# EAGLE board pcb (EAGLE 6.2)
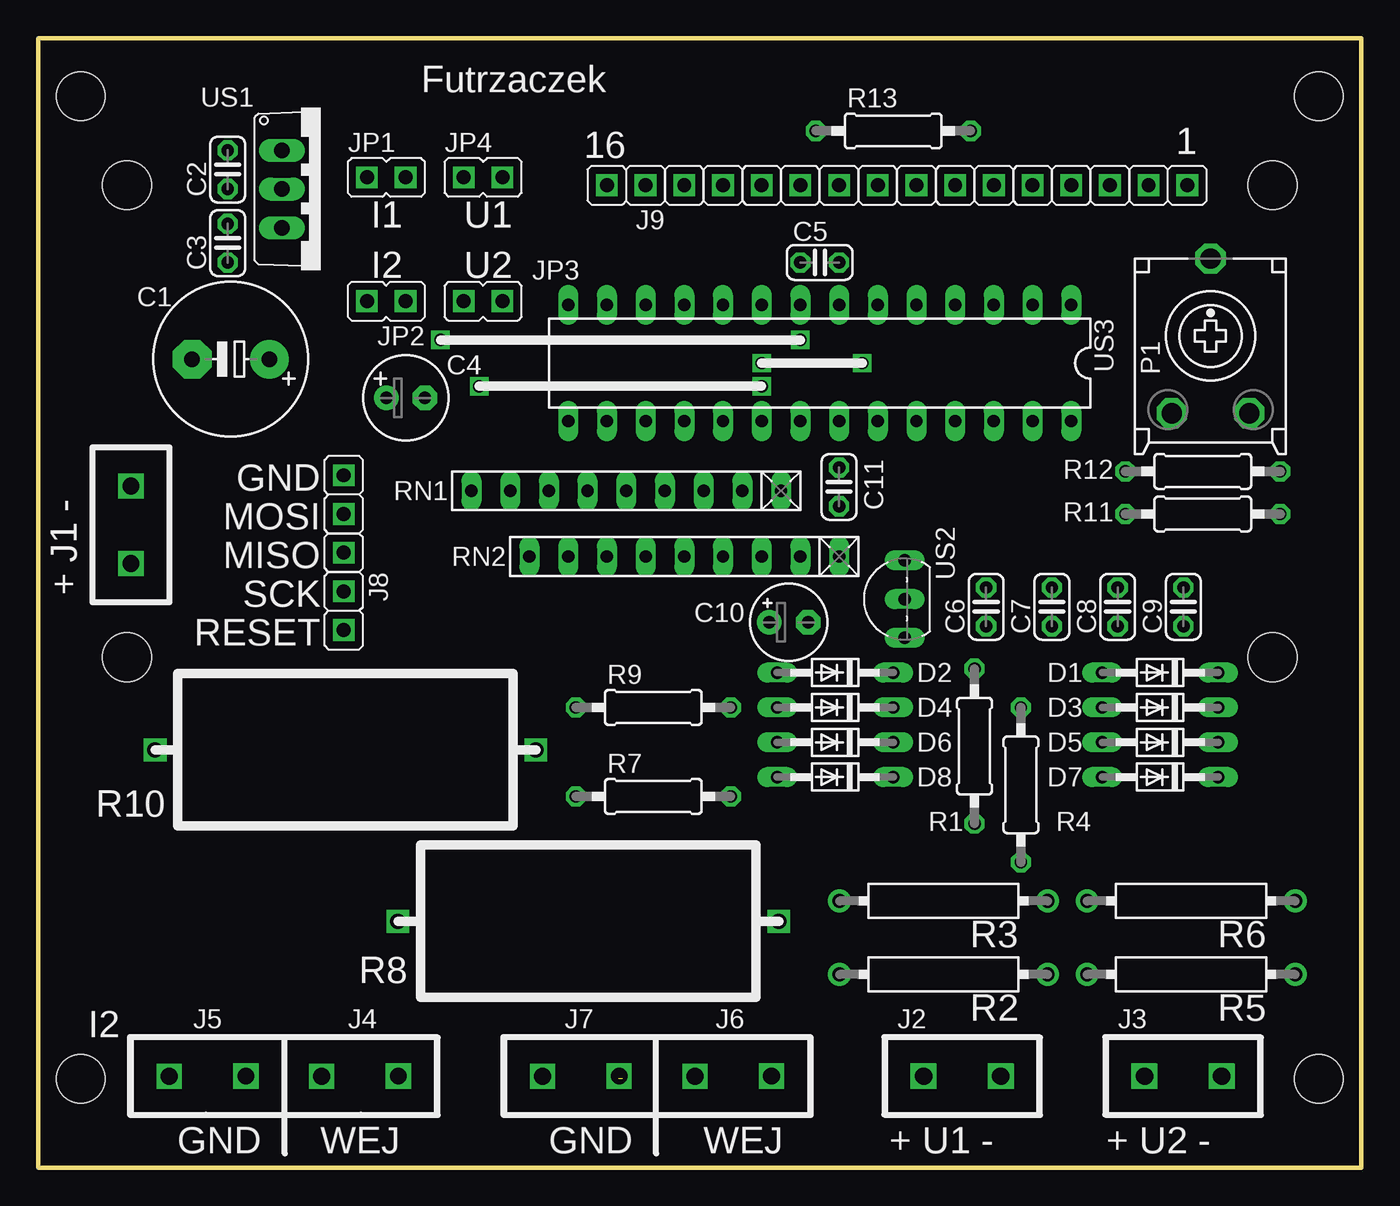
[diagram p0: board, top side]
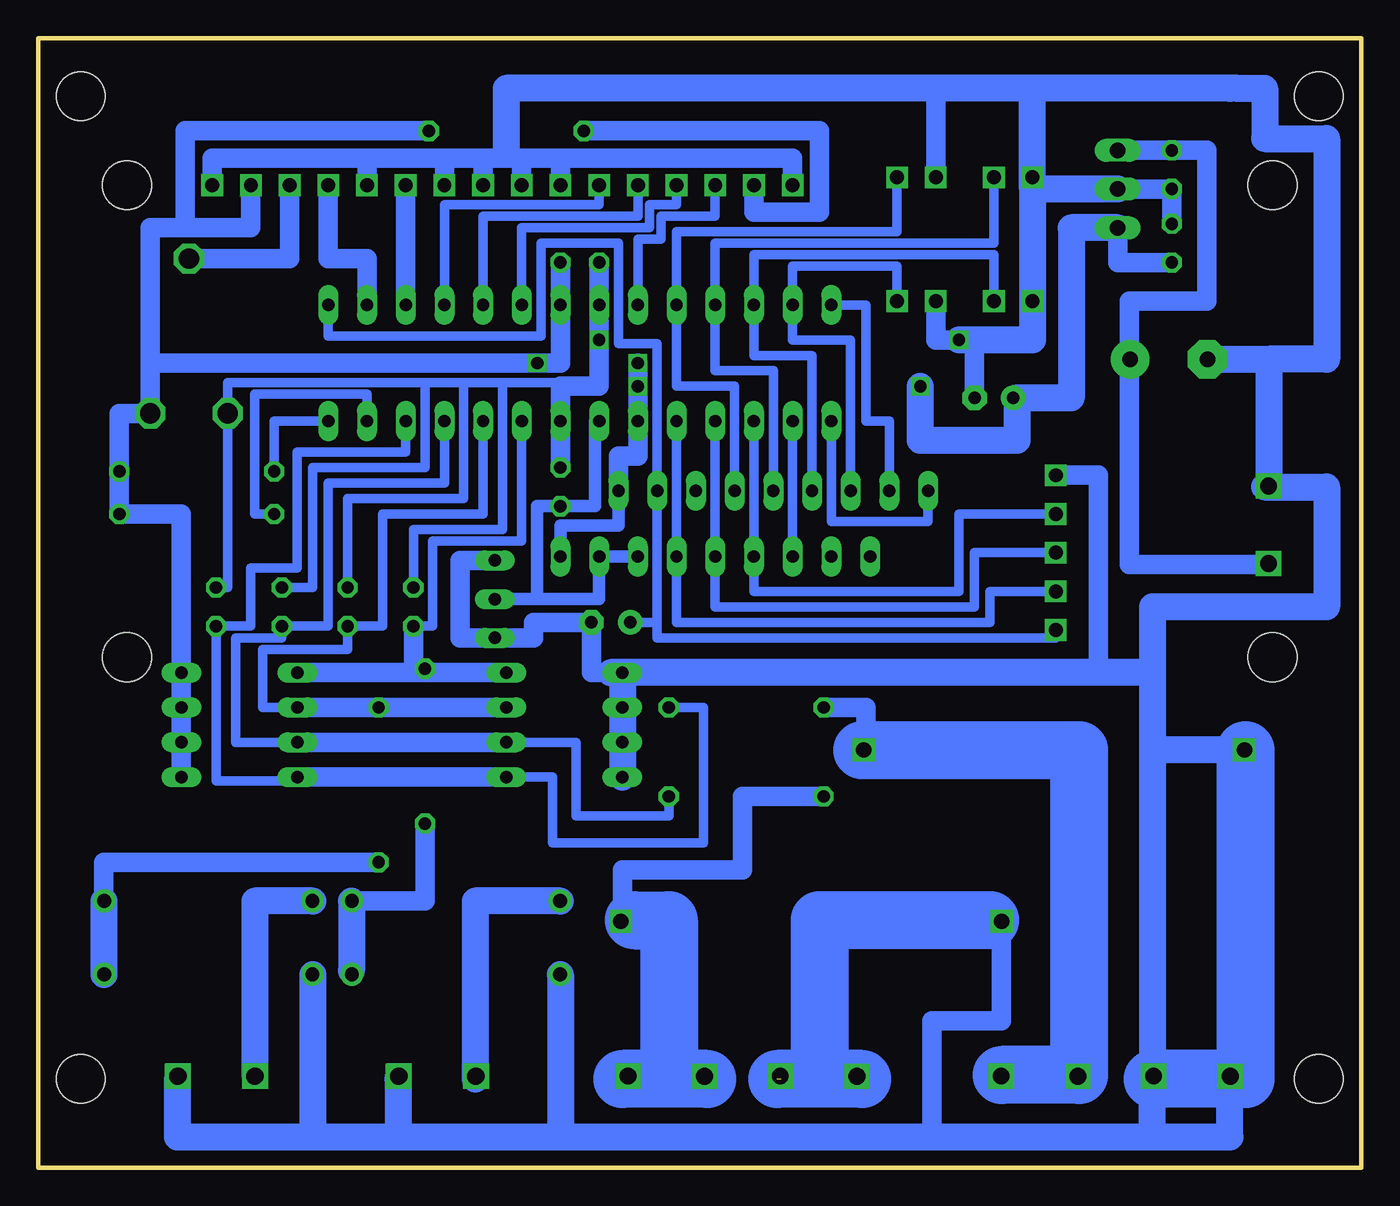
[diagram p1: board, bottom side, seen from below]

Size 86.87 x 74.17 mm. Coordinates in mm from the lower left corner, seen from the top.
Outline: 0,74.17 0,0 86.87,0 86.87,74.17 0,74.17
Copper layers (1*16): Top 0.035mm / dielectric 1.5mm / Bottom 0.035mm
Design rules: minimum track width 10mil, minimum drill 24mil, track to track 8mil, track to pad 8mil, pad to pad 8mil, via to via 8mil, smd to smd 8mil, copper to edge 40mil, drill to drill 8mil, minimum pad ring 10mil, minimum via ring 8mil, stop-mask expansion 4mil, vias tented up to drill 0mil, thermal gap 10mil
Holes 3.2 mm at 5.84,33.53 5.84,64.52 81.03,64.52 81.03,33.53 2.79,5.84 84.07,5.84 2.79,70.36 84.07,70.36

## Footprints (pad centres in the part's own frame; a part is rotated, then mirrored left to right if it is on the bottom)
E5-10,5 = drill 1.016 pad 2.54: + -2.54,0 | drill 1.016 pad 2.54 octagon: - 2.54,0
C025-024X044 = drill 0.813 octagon: 1 -1.27,0; 2 1.27,0
E2,5-6 = drill 0.813 pad 1.6: + -1.27,0 | drill 0.813 pad 1.6 octagon: - 1.27,0
E2,5-5 = drill 0.813 pad 1.6: + -1.27,0 | drill 0.813 pad 1.6 octagon: - 1.27,0
DO34-7 = drill 0.813 long: A 3.81,0; C -3.81,0
JP1 = drill 0.914 pad 1.422 square: 1 0,-1.27; 2 0,1.27
ECP10S = drill 1.321 octagon: A -2.54,-5.08; E 2.54,-5.08; S 0,5.08
0207/10 = drill 0.813 octagon: 1 -5.08,0; 2 5.08,0
HPS63 = drill 0.9 pad 1.5: 1 -6.83,0; 2 6.83,0
RN-9 = drill 0.813 long: 1 -10.16,0; 2 -7.62,0; 3 -5.08,0; 4 -2.54,0; 5 0,0; 6 2.54,0; 7 5.08,0; 8 7.62,0; 9 10.16,0
TO220V = drill 1.016 long: 1 -2.54,-2.54; 2 0,-2.54; 3 2.54,-2.54
TO92- = drill 0.813 long: 1 2.54,0; 2 0,0; 3 -2.54,0
DIL28-3 = drill 0.813 long: 1 -16.51,-3.81; 2 -13.97,-3.81; 3 -11.43,-3.81; 4 -8.89,-3.81; 5 -6.35,-3.81; 6 -3.81,-3.81; 7 -1.27,-3.81; 8 1.27,-3.81; 9 3.81,-3.81; 10 6.35,-3.81; 11 8.89,-3.81; 12 11.43,-3.81; 13 13.97,-3.81; 14 16.51,-3.81; 15 16.51,3.81; 16 13.97,3.81; 17 11.43,3.81; 18 8.89,3.81; 19 6.35,3.81; 20 3.81,3.81; 21 1.27,3.81; 22 -1.27,3.81; 23 -3.81,3.81; 24 -6.35,3.81; 25 -8.89,3.81; 26 -11.43,3.81; 27 -13.97,3.81; 28 -16.51,3.81

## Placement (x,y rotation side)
C1  [E5-10,5]  12.65,53.09 180 top
C2  [C025-024X044]  12.45,65.53 90 top
C3  [C025-024X044]  12.45,60.71 90 top
C4  [E2,5-6]  24.13,50.55 0 top
C5  [C025-024X044]  51.31,59.44 0 top
C6  [C025-024X044]  62.23,36.83 90 top
C7  [C025-024X044]  66.55,36.83 90 top
C8  [C025-024X044]  70.87,36.83 90 top
C9  [C025-024X044]  75.18,36.83 90 top
C10  [E2,5-5]  49.28,35.81 0 top
C11  [C025-024X044]  52.58,44.7 90 top
D1  [DO34-7]  73.66,32.51 180 top
D2  [DO34-7]  52.32,32.51 180 top
D3  [DO34-7]  73.66,30.23 180 top
D4  [DO34-7]  52.32,30.23 180 top
D5  [DO34-7]  73.66,27.94 180 top
D6  [DO34-7]  52.32,27.94 180 top
D7  [DO34-7]  73.66,25.65 180 top
D8  [DO34-7]  52.32,25.65 180 top
E$3  [JP1]  41.15,64.52 90 top
E$4  [JP1]  43.69,64.52 90 top
E$5  [JP1]  46.23,64.52 90 top
E$6  [JP1]  48.77,64.52 90 top
E$7  [JP1]  51.31,64.52 90 top
E$8  [JP1]  53.85,64.52 90 top
E$9  [JP1]  56.39,64.52 90 top
E$10  [JP1]  58.93,64.52 90 top
E$11  [JP1]  61.47,64.52 90 top
E$12  [JP1]  64.01,64.52 90 top
E$13  [JP1]  66.55,64.52 90 top
E$14  [JP1]  69.09,64.52 90 top
E$15  [JP1]  71.63,64.52 90 top
E$16  [JP1]  74.17,64.52 90 top
E$23  [JP1]  20.07,39.12 180 top
E$25  [JP1]  20.07,41.66 180 top
E$26  [JP1]  20.07,44.2 180 top
J8  [JP1]  20.07,36.58 180 top
J9  [JP1]  38.61,64.52 90 top
JP1  [JP1]  22.86,65.02 270 top
JP2  [JP1]  22.86,56.9 90 top
JP3  [JP1]  29.21,56.9 90 top
JP4  [JP1]  29.21,65.02 270 top
P1  [ECP10S]  76.96,54.61 0 top
R1  [0207/10]  61.47,27.69 270 top
R2  [HPS63]  59.44,12.7 180 top
R3  [HPS63]  59.44,17.53 180 top
R4  [0207/10]  64.52,25.15 270 top
R5  [HPS63]  75.69,12.7 180 top
R6  [HPS63]  75.69,17.53 180 top
R7  [0207/10]  40.39,24.38 0 top
R9  [0207/10]  40.39,30.23 0 top
R11  [0207/10]  76.45,42.93 180 top
R12  [0207/10]  76.45,45.72 180 top
R13  [0207/10]  56.13,68.07 0 top
RN1  [RN-9]  38.61,44.45 180 top
RN2  [RN-9]  42.42,40.13 180 top
US1  [TO220V]  18.54,64.26 270 top
US2  [TO92-]  56.9,37.34 90 top
US3  [DIL28-3]  51.31,52.83 180 top

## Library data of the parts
C1-C11 R1 R4 R7 R9 R11-R13 = rcl
D1-D8 = diode
E$3-E$16 E$23 E$25 E$26 J8 J9 JP1-JP4 = hybrid
P1 = pot
R2 R3 R5 R6 = resistor-power
RN1 RN2 = resistor-net
US1 US2 = transistor-npn
US3 = 40xx

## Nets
S$2: US3.9
S$3: E$7.1 E$8.1 E$9.1 E$10.1 E$12.1 E$16.1 J9.2
S$4: C10.+ J8.2 RN1.2 US3.1
S$6: R9.1
S$7: J9.1 R13.1
S$8: E$14.1
S$9: E$13.1 US3.2
S$10: E$11.1 US3.3
S$11: E$6.1 US3.4
S$12: E$5.1 US3.5
S$14: RN1.1 RN2.1 US3.20
S$15: US3.21
S$16: US3.6
S$17: RN1.9 US3.15
S$18: RN1.8 US3.14
S$22: C5.2 D7.C E$15.1 P1.E R11.1 R13.2 US3.7
S$23: JP1.2 RN1.5 US3.11
S$24: JP2.1 RN1.6 US3.12
S$26: JP3.1 RN1.7
S$27: R7.1
S$28: C3.1 US1.3
S$29: C10.- D8.A E$26.1 US2.1 US2.3
S$30: JP4.2 RN1.4 US3.10
S$31: J8.1 RN2.4 US3.19
S$32: RN2.5 US3.18
S$33: E$25.1 RN2.6 US3.17
S$34: RN2.7 US3.16
S$35: R11.2 US3.27
S$62: C5.1 C6.2 C7.2 C8.2 C9.2 P1.A US3.8 US3.22
S$86: C2.2 US1.1
S$97: R12.2 US3.28
S$98: C6.1 D1.A D2.C
S$99: C9.1 US3.26
S$101: C7.1 D3.A D4.C US3.24
S$104: C3.2 C4.- JP3.2 JP4.1 US1.2
S$111: C8.1 D5.A D6.C R7.2 US3.25
S$112: D7.A R9.2
S$114: R4.2
S$115: R1.2

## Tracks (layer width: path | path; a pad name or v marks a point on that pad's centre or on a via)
S$1
  Bottom 3.81: 42.93,5.84 48.51,5.84
S$2
  Bottom 0.61: 42.42,64.26 42.42,62.48 45.97,62.48 45.97,60.96 47.5,60.96 US3.9
S$3
  Bottom 1.27: E$16.1 75.44,66.29 65.28,66.29 | 65.28,66.29 E$12.1 | 65.28,66.29 60.2,66.29 | 60.2,66.29 E$10.1 | 60.2,66.29 57.66,66.29 | 57.66,66.29 E$9.1 | 57.66,66.29 55.12,66.29 | 55.12,66.29 E$8.1 | 55.12,66.29 52.58,66.29 | 52.58,66.29 E$7.1 | 52.58,66.29 37.34,66.29 J9.2
S$4
  Bottom 0.61: US3.1 67.82,54.61 53.85,54.61 53.85,60.71 48.77,60.71 48.77,54.1 46.23,54.1 RN1.2 46.23,35.81 | 46.23,35.81 46.23,34.8 20.07,34.8 J8.2 | C10.+ 46.23,35.81
S$5
  Bottom 1.27: 43.18,6.1 45.47,6.1 | 45.47,6.1 48.26,6.1 | 45.47,6.1 45.47,6.35
  Bottom 3.81: 47.75,16.26 45.47,16.26 45.47,6.35
S$6
  Bottom 1.27: 18.54,27.43 32.51,27.43 32.51,30.23 R9.1
  Bottom 3.81: 32.77,27.43 18.54,27.43 18.54,6.1 23.62,6.1
S$7
  Bottom 1.27: J9.1 39.88,62.74 35.56,62.74 35.56,68.07 R13.1
S$8
  Bottom 1.27: 77.22,59.69 70.36,59.69 E$14.1
S$9
  Bottom 1.27: US3.2 65.28,59.69 67.82,59.69 E$13.1
S$10
  Bottom 1.27: US3.3 E$11.1
S$11
  Bottom 0.61: E$6.1 50.04,63.25 60.2,63.25 US3.4
S$12
  Bottom 0.61: E$5.1 47.5,62.48 57.66,62.48 US3.5
S$13
  Bottom 1.27: 38.1,6.1 35.56,6.1 33.02,6.1
  Bottom 3.81: 24.38,16.26 35.56,16.26 35.56,6.1
S$14  (via drill 0.8)
  Bottom 0.813: RN2.1 52.58,42.16 48.77,42.16 RN1.1
  Bottom 1.27: RN1.1 48.77,46.74 47.5,46.74 US3.20 v47.5,51.31 v47.5,52.83
S$15
  Bottom 0.813: 47.24,40.13 50.04,40.13 50.04,37.34 54.1,37.34 | 54.1,37.34 56.9,37.34 | 54.1,37.34 54.1,43.43 50.29,43.43 50.29,49.02 US3.21
S$16
  Bottom 0.61: 44.96,64.26 44.96,63.25 46.74,63.25 46.74,61.72 55.12,61.72 US3.6
S$17
  Bottom 0.61: RN1.9 28.45,42.42 34.8,42.42 US3.15
S$18
  Bottom 0.61: US3.14 32.51,56.64 32.51,49.02 30.99,49.02 RN1.8
S$19  (1 unrouted)
  Bottom 3.81: 32.77,5.84 38.35,5.84
S$20  (via drill 1.1)
  other vias: 6.1,44.75
S$21  (via drill 1.1)
  other vias: 6.1,39.67
S$22  (via drill 0.8)
  Bottom 1.27: C5.2 US3.7 52.58,52.83 v54.1,52.83 79.5,52.83 | E$15.1 72.9,61.72 77.22,61.72 | 77.22,61.72 79.5,61.72 79.5,52.83 | 79.5,52.83 P1.E 81.53,49.53 R11.1 77.47,42.93 D7.C | R13.2 77.22,68.07 77.22,61.72
S$23
  Bottom 0.61: JP1.2 24.13,60.71 42.42,60.71 US3.11 42.42,52.32 38.61,52.32 RN1.5
S$24
  Bottom 0.61: JP2.1 24.13,59.94 39.88,59.94 US3.12 39.88,53.34 36.07,53.34 RN1.6
S$25
  Bottom 1.27: 23.62,16 23.62,9.65 28.19,9.65 28.19,2.29
S$26
  Bottom 0.61: JP3.1 30.48,59.18 37.34,59.18 37.34,54.36 33.53,54.36 RN1.7
S$27
  Bottom 1.27: R7.1 40.64,24.38 40.64,19.56 48.51,19.56 48.51,16.26
S$28  (via drill 0.8)
  Bottom 1.27: 28.96,47.75 22.86,47.75 22.86,50.55 19.05,50.55 | C3.1 16,59.44 US1.3
  Bottom 1.778: US1.3 19.05,61.72 19.05,50.55 22.61,50.55 22.61,47.75 28.96,47.75 v28.96,51.31
S$29
  Bottom 1.27: 13.46,6.1 8.64,6.1 | 8.64,6.1 7.62,6.1 7.62,27.43 | 68.83,2.03 63.25,2.03 | 63.25,2.03 63.25,2.29 | 63.25,5.84 63.25,6.1 | 63.25,2.03 52.58,2.03 | 52.58,2.03 38.1,2.03 | 33.02,2.03 13.72,2.03 | 13.72,4.32 13.72,5.59 13.72,5.84 13.72,32.51 13.97,32.51 17.27,32.51 | E$26.1 17.27,45.47 17.27,32.51 | 17.27,32.51 48.51,32.51 | 49.28,32.51 50.55,32.51 C10.- 54.36,35.81 54.36,34.8 US2.3 59.18,34.8 59.18,39.88 US2.1 | 8.64,6.1 8.64,4.32 | 52.58,2.29 52.58,2.03 | 13.21,27.43 13.46,27.43
  Bottom 1.778: 6.35,44.7 2.29,44.7 2.29,36.83 13.72,36.83 13.72,5.59 | 77.72,5.84 77.72,2.03 68.83,2.03 | 68.83,2.03 38.1,2.03 33.02,2.03 8.64,2.03 8.64,4.32 | 13.72,2.03 13.72,4.32 | 63.25,5.84 63.25,2.29 | 52.58,12.7 52.58,2.29 | 68.83,12.7 68.83,2.03 | 7.62,27.43 13.21,27.43 | 13.97,32.51 48.51,32.51 | 48.51,32.51 49.28,32.51 | 48.51,32.51 D8.A
  Bottom 3.81: 7.62,27.43 7.62,5.84 13.72,5.84
S$30
  Bottom 0.61: RN1.4 41.15,51.31 44.96,51.31 US3.10 44.96,61.47 30.48,61.47 JP4.2
S$31
  Bottom 0.61: US3.19 RN2.4 44.96,35.81 24.38,35.81 24.38,37.85 J8.1
S$32
  Bottom 0.61: US3.18 RN2.5 42.42,36.83 25.4,36.83 25.4,40.39 20.07,40.39
S$33
  Bottom 0.61: US3.17 RN2.6 39.88,37.85 26.42,37.85 26.42,42.93 E$25.1
S$34
  Bottom 0.61: US3.16 RN2.7
S$35
  Bottom 0.61: US3.27 65.28,50.8 72.64,50.8 72.64,42.93 R11.2
S$38  (via drill 1.1)
  other vias: 58.14,6.02
S$39  (via drill 1.1)
  other vias: 63.22,6.02
S$44  (via drill 1.1)
  other vias: 58.1,6.03
S$45  (via drill 1.1)
  other vias: 63.18,6.03
S$54  (via drill 1.1)
  other vias: 58.14,6.02
S$55  (via drill 1.1)
  other vias: 63.22,6.02
S$56  (via drill 1.1)
  other vias: 72.64,6.02
S$62  (via drill 0.8)
  Bottom 0.61: C8.2 68.83,38.1 68.83,45.97 61.47,45.97 61.47,51.56 | C6.2 62.23,41.91 56.39,41.91 56.39,51.56 | 61.47,51.56 74.42,51.56 P1.A 74.42,38.1 C9.2 | 61.47,51.56 58.93,51.56 | 58.93,51.56 56.39,51.56 | 56.39,51.56 52.58,51.56 52.58,50.55 | 58.93,51.56 58.93,43.94 66.55,43.94 C7.2
  Bottom 1.27: C5.1 US3.8 v50.04,54.36 50.04,51.31 52.58,51.31 52.58,50.55 US3.22 52.58,45.97
S$67  (via drill 1.1)
  other vias: 8.61,6.02
S$68  (via drill 1.1)
  other vias: 13.65,6.03
S$71  (via drill 1.1)
  other vias: 18.61,6.02
S$72  (via drill 1.1)
  other vias: 23.65,6.03
S$76  (via drill 1)
  other vias: 7.68,27.44
S$77  (via drill 1)
  other vias: 32.68,27.44
S$78  (via drill 1.1)
  other vias: 33.11,6.02
S$79  (via drill 1.1)
  other vias: 38.15,6.03
S$80  (via drill 1.1)
  other vias: 43.11,6.02
S$81  (via drill 1.1)
  other vias: 48.15,6.03
S$82  (via drill 1)
  other vias: 23.62,16.19
S$86
  Bottom 1.27: 6.1,39.62 15.24,39.62 15.24,56.9 10.16,56.9 10.16,66.8 C2.2 US1.1
S$97
  Bottom 0.61: US3.28 71.37,49.02 R12.2
S$98
  Bottom 0.61: 55.12,49.02 55.12,41.15 60.96,41.15 60.96,35.56 C6.1
  Bottom 1.27: D2.C 62.23,32.51 | 62.23,32.51 D1.A | C6.1 62.23,32.51
S$99
  Bottom 0.61: US3.26 62.74,46.99 69.85,46.99 69.85,39.37 72.9,39.37 72.9,35.56 C9.1 75.18,25.4 69.85,25.4
S$101
  Bottom 0.61: US3.24 57.66,42.93 64.26,42.93 64.26,35.56 C7.1 66.55,34.04 72.14,34.04 72.14,30.23 D3.A
  Bottom 1.27: D3.A D4.C
S$102  (via drill 1)
  other vias: 48.62,16.19
S$103  (via drill 1.1)
  other vias: 77.72,6.02
S$104  (via drill 0.8)
  Bottom 1.27: US1.2 12.45,64.26 C3.2 | 56.39,66.55 56.13,66.55 56.13,67.06 | 56.13,70.87 27.94,70.87 | 27.94,70.87 JP4.1 | 27.94,70.87 21.59,70.87 | 21.59,70.87 21.59,70.36 | 21.59,54.36 25.4,54.36 | 25.4,54.36 v26.42,54.36 27.94,54.36 JP3.2 | 21.59,70.87 8.64,70.87 | 8.13,70.87 7.87,70.87 | C4.- 25.4,54.36
  Bottom 1.778: 56.13,67.06 56.13,70.87 8.64,70.87 8.13,70.87 6.35,70.87 6.35,67.56 2.29,67.56 2.29,53.09 6.1,53.09 | 10.16,53.09 6.1,53.09 | 6.1,53.09 6.1,44.7 | US1.2 21.59,64.26 | 21.59,64.26 21.59,70.36 | 21.59,64.26 21.59,54.36 v26.42,54.36
S$105  (via drill 1.1)
  other vias: 72.64,6.02
S$108  (via drill 1.1)
  other vias: 77.72,6.02
S$109  (via drill 1.1)
  other vias: 72.6,6.03
S$110  (via drill 1.1)
  other vias: 77.68,6.03
S$111
  Bottom 0.61: R7.2 45.47,23.11 51.56,23.11 51.56,27.94 D6.C | D5.A 73.91,27.94 73.91,34.8 70.87,34.8 C8.1 67.82,35.56 67.82,44.96 60.2,44.96 US3.25
  Bottom 1.27: D6.C D5.A
S$112
  Bottom 0.61: R9.2 43.18,30.23 43.18,21.34 53.09,21.34 53.09,25.65 56.13,25.65
  Bottom 1.27: D7.A 56.13,25.65 55.88,25.65
S$114
  Bottom 1.27: 82.55,17.53 82.55,20.07 R4.2
  Bottom 1.778: 82.55,17.53 82.55,12.7
S$115
  Bottom 1.27: 66.29,12.95 66.29,12.7 | 66.29,17.53 61.47,17.53 R1.2
  Bottom 1.778: 66.29,17.53 66.29,12.95
S$116
  Bottom 1.27: 58.17,17.53 58.17,6.1
  Bottom 1.778: 52.58,17.53 58.17,17.53 58.17,5.84
S$117
  Bottom 1.778: 68.83,17.53 72.64,17.53 72.64,6.1

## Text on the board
tPlace: + J1 - | I2 | GND | WEJ | GND | WEJ | + U1 - | + U2 -
tNames: Futrzaczek | 1 | 16 | I1 | U1 | I2 | U2 | GND | MOSI | MISO | SCK | RESET | R10 | R8 | J5 | J4 | J7 | J6 | J2 | J3
tValues: I1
